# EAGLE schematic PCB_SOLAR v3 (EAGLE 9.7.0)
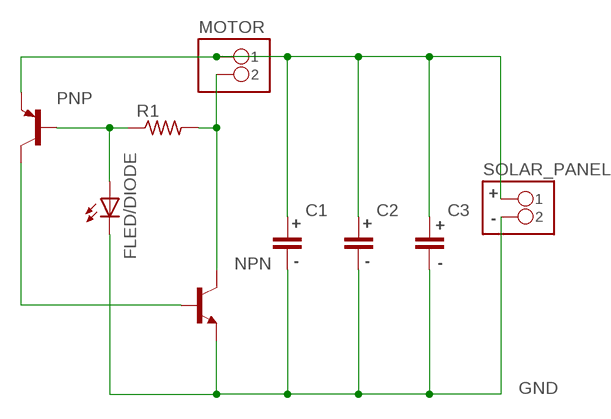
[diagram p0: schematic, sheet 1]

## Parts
C1  C_RADIAL-12.5MM-DIA  [CAPRD550W60D1025H1250B]
C2  C_RADIAL-12.5MM-DIA  [CAPRD550W60D1025H1250B]
C3  C_RADIAL-12.5MM-DIA  [CAPRD550W60D1025H1250B]
FLED/DIODE  LED5MM  [LED5MM]
MOTOR  PINHD-1X02_1X02M  [1X02]
NPN  2N2222  [TO92-EBC-OVAL]
PNP  2N2907  [TO92-EBC-OVAL]
R1  R-US_AXIAL-7.2MM-PITCH  [RESAD724W46L381D178B]
SOLAR_PANEL  PINHD-1X02_1X02M  [1X02]

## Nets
GND: C1.2 C2.2 C3.2 FLED/DIODE.K(C) NPN.E SOLAR_PANEL.2
N$1: FLED/DIODE.A PNP.B R1.1
N$2: C1.1 C2.1 C3.1 MOTOR.1 PNP.E SOLAR_PANEL.1
N$3: MOTOR.2 NPN.C R1.2
N$5: NPN.B PNP.C

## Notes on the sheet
- +
- -
- + | + | +
- - | - | -

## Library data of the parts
C1-C3 = Tutorial - Fusion 360:C: Capacitor - Generic; CATEGORY: Capacitor
FLED/DIODE = Library:LED: LED
MOTOR SOLAR_PANEL = Tinkercad:PINHD-1X02
NPN = Library:2N2222: NPN TRANSISTOR Big oval pads
PNP = Library:2N2907*: PNP Transistor Big Oval pads
R1 = Tutorial - Fusion 360:R-US: Resistor Fixed - ANSI; CATEGORY: Resistor; SUB-CATEGORY: Fixed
